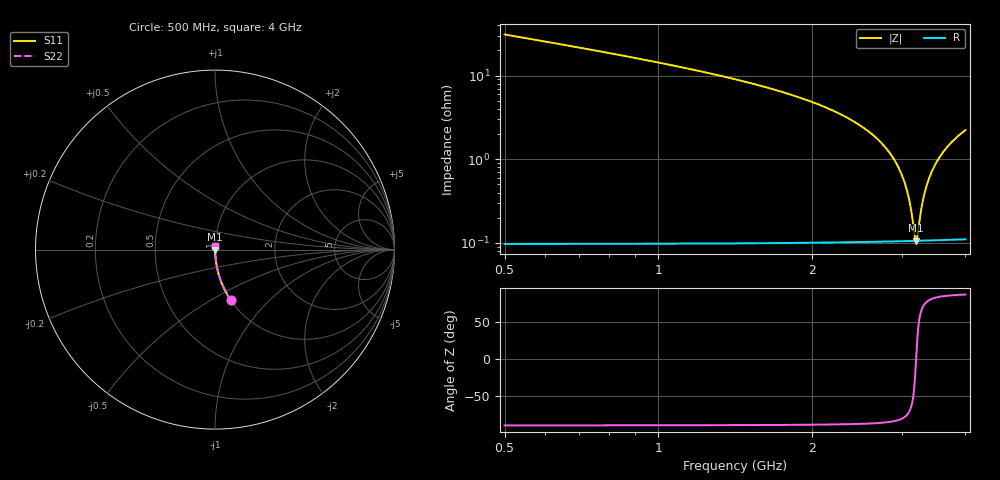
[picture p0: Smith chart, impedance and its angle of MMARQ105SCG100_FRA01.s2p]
! MMARQ105SCG100_FRA01  S-PARAMETER MODEL  ( General Type )
! Model Generated by TAIYO YUDEN Corporation (http://www.ty-top.com)
! Version 1.0
! TAIYO YUDEN Control No. 200326
! Copyright(c) 2020 TAIYO YUDEN CO.,LTD. All Rights Reserved.
! Product Description (link to TY-COMPAS)
! https://ds.yuden.co.jp/TYCOMPAS/or/detail?pn=MMARQ105SCG100JFRA01&u=M
! Products Name : Multilayer Ceramic Capacitors
! Characteristics :
!  Capacitance : 10 pF , Rated Voltage : 250V , TCC : CG / C0G
!  Case Size : 1.0 x 0.5 / 0.039 x 0.02 [mm/inch] , Thickness : 0.5 / 0.02 [mm/inch]
!  (Conditions: Temperature = 25 degC , DC Bias Current/Voltage = 0A / 0V)
! External Node Assignments :
!  1  o---| |---o  2
! GND o---------o GND
! Frequency Range : 500MHz  -  4GHz  [ 401 STEP ]
# MHz S RI R 50
! Freq[MHz].  S11 Real  S11 Imag  S21 Real  S21 Imag  S12 Real  S12 Imag  S22 Real  S22 Imag
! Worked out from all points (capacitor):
!   401 points, 500 MHz to 4 GHz, reference 50 ohm
!   read as one part in series: C = 10 pF near 517.5 MHz
!   lowest |Z| = 106 mohm at 3.204 GHz (marker M1)
!   series resonance near 3.202 GHz, so ESL is about 250 pH
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500  0.0886 -0.2826  0.9114 0.2826  0.9114 0.2826  0.0886 -0.2826
753.75  0.0391 -0.1914  0.9609 0.1914  0.9609 0.1914  0.0391 -0.1914
1086.25  0.0174 -0.1272  0.9826 0.1272  0.9826 0.1272  0.0174 -0.1272
1672.5  0.00574 -0.0687  0.9943 0.0687  0.9943 0.0687  0.00574 -0.0687
2250  0.00229 -0.0357  0.9977 0.0357  0.9977 0.0357  0.00229 -0.0357
2591.25  0.00147 -0.0211  0.9985 0.0211  0.9985 0.0211  0.00147 -0.0211
2836.25  0.00118 -0.0121  0.9988 0.0121  0.9988 0.0121  0.00118 -0.0121
2958.75  0.00111 -0.00785  0.9989 0.00785  0.9989 0.00785  0.00111 -0.00785
3046.25  0.00107 -0.00496  0.9989 0.00496  0.9989 0.00496  0.00107 -0.00496
3107.5  0.00106 -0.00298  0.9989 0.00298  0.9989 0.00298  0.00106 -0.00298
3133.75  0.00106 -0.00215  0.9989 0.00215  0.9989 0.00215  0.00106 -0.00215
3186.25  0.00106 -0.000502  0.9989 0.000502  0.9989 0.000502  0.00106 -0.000502
3203.75  0.00106 4.05e-05  0.9989 -4.05e-05  0.9989 -4.05e-05  0.00106 4.05e-05
3221.25  0.00106 0.00058  0.9989 -0.00058  0.9989 -0.00058  0.00106 0.00058
3273.75  0.00106 0.00218  0.9989 -0.00218  0.9989 -0.00218  0.00106 0.00218
3308.75  0.00107 0.00324  0.9989 -0.00324  0.9989 -0.00324  0.00107 0.00324
3361.25  0.00109 0.0048  0.9989 -0.0048  0.9989 -0.0048  0.00109 0.0048
3422.5  0.00111 0.00659  0.9989 -0.00659  0.9989 -0.00659  0.00111 0.00659
3527.5  0.00117 0.00959  0.9988 -0.00959  0.9988 -0.00959  0.00117 0.00959
3650  0.00125 0.013  0.9987 -0.013  0.9987 -0.013  0.00125 0.013
3816.25  0.0014 0.0175  0.9986 -0.0175  0.9986 -0.0175  0.0014 0.0175
4000  0.0016 0.0222  0.9984 -0.0222  0.9984 -0.0222  0.0016 0.0222
